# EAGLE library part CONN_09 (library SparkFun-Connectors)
Multi connection point. Often used as Generic Header-pin footprint for 0.1 inch spaced/style header connections On any of the 0.1 inch spaced packages, you can populate with these: Break Away Headers - Straight (PRT-00116) Break Away Male Headers - Right Angle (PRT-00553) Female Headers (PRT-00115) Break Away Headers - Machine Pin (PRT-00117) Break Away Female Headers - Swiss Machine Pin (PRT-00743) For SCREWTERMINALS and SPRING TERMINALS visit here: Screw Terimnals on SparkFun.com (5mm/3.5mm/2.54mm spacing) This device is also useful as a general connection point to wire up your design to another part of your project. Our various solder wires solder well into these plated through hole pads. Hook-Up Wire - Assortment (Stranded, 22 AWG) (PRT-11375) Hook-Up Wire - Assortment (Solid Core, 22 AWG) (PRT-11367) View the entire wire category on our website here Special notes: Molex polarized connector foot print use with SKU : PRT-08231 with associated crimp pins and housings. 1MM SMD Version SKU: PRT-10208 NOTES ON THE VARIANTS LOCK and LOCK_LONGPADS... This footprint was designed to help hold the alignment of a through-hole component (i.e. 6-pin header) while soldering it into place. You may notice that each hole has been shifted either up or down by 0.005 of an inch from it's more standard position (which is a perfectly straight line). This slight alteration caused the pins (the squares in the middle) to touch the edges of the holes. Because they are alternating, it causes a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
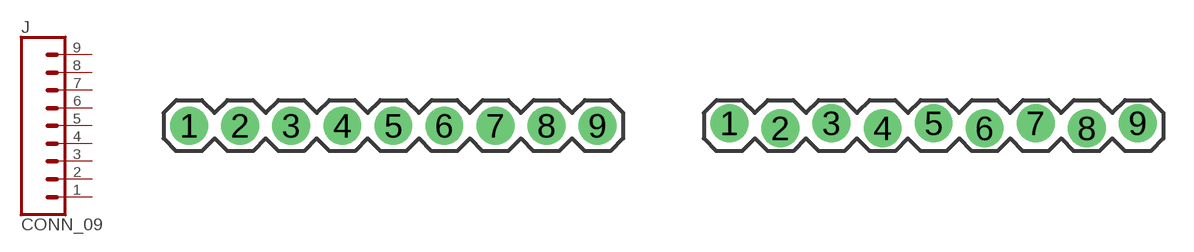
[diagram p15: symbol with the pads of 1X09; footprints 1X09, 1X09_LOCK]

Designator prefix J

## CONN_09  [1X09]
1  1  pas
2  2  pas
3  3  pas
4  4  pas
5  5  pas
6  6  pas
7  7  pas
8  8  pas
9  9  pas

## CONN_09LOCK  [1X09_LOCK]
Pads as for 1X09

## CONN_09LOCK-LONGPADS  [1X09_LOCK_LONGPADS]
Pads as for 1X09

## CONN_09LONGPADS  [1X09_LONGPADS]
Pads as for 1X09

## CONN_09NO_SILK  [1X09_NO_SILK]
Pads as for 1X09

## CONN_093.5MM-9  [SCREWTERMINAL-3.5MM-9]
Pads as for 1X09

## Footprint 1X09 (pad centres in mm)
Plated Through Hole -9 Pin Specifications: Pin count:9 Pin pitch:0.1" Example device(s): CONN_09
drill 1.016 pad 1.88: 1 0,0; 2 2.54,0; 3 5.08,0; 4 7.62,0; 5 10.16,0; 6 12.7,0; 7 15.24,0; 8 17.78,0; 9 20.32,0

## Footprint 1X09_LOCK (pad centres in mm)
Plated Through Hole -9 Pin Locking Footprint Holes are offset 0.005" to lock pins in place during soldering. Specifications: Pin count:9 Pin pitch:0.1" Example device(s): CONN_09
drill 1.016 pad 1.88: 1 0,0.127; 2 2.54,-0.127; 3 5.08,0.127; 4 7.62,-0.127; 5 10.16,0.127; 6 12.7,-0.127; 7 15.24,0.127; 8 17.78,-0.127; 9 20.32,0.127

## Footprint 1X09_LOCK_LONGPADS (pad centres in mm)
Plated Through Hole -9 Pin Locking Footprint w/ Long Pads Holes are offset 0.005" to lock pins in place during soldering. Specifications: Pin count:9 Pin pitch:0.1" Example device(s): CONN_09
drill 1.016 long: 1 0,0.127; 2 2.54,-0.127; 3 5.08,0.127; 4 7.62,-0.127; 5 10.16,0.127; 6 12.7,-0.127; 7 15.24,0.127; 8 17.78,-0.127; 9 20.32,0.127

## Footprint 1X09_LONGPADS (pad centres in mm)
Plated Through Hole -9 Pin Long Pads Specifications: Pin count:9 Pin pitch:0.1" Example device(s): CONN_09
drill 1.118 pad 1.88 long: 1 0,0; 2 2.54,0; 3 5.08,0; 4 7.62,0; 5 10.16,0; 6 12.7,0; 7 15.24,0; 8 17.78,0; 9 20.32,0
